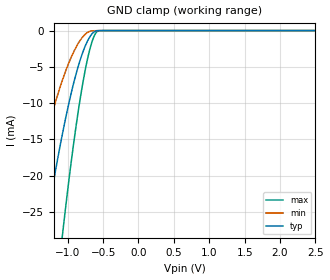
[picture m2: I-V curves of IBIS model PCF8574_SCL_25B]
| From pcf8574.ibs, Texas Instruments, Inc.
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[Model]   PCF8574_SCL_25B
Model_type  Input
Vinl=.75
Vinh=1.75
| variable   typ   min   max
C_comp   1.04pF   0.96pF   1.20pF
[Temperature Range]   40   100   -40
| Ambient temperature   25   85   -40
[Voltage range]   2.5   2.5   2.5
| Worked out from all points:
|   GND clamp passes 1 mA (typ) near -0.70 V on its own axis
[GND Clamp]
| PCF8574_SCL_25B
|   Voltage   I(typ)   I(min)   I(max)
-2.5V     -117.1mA   -74.13mA   -195.1mA
-1.63V    -48.43mA   -28.12mA   -85.63mA
-1.6V     -46.32mA   -26.75mA   -82.18mA
-1.315V   -27.58mA   -14.86mA   -51.15mA
-1.07V    -14.04mA   -6.717mA   -27.86mA
-960mV    -9.033mA   -3.902mA   -18.86mA
-870mV    -5.578mA   -2.087mA   -12.39mA
-790mV    -3.09mA    -907.2uA   -7.454mA
-710mV    -1.254mA   -201.3uA   -3.496mA
-630mV    -200.9uA   -23.45uA   -857.1uA
-560mV    -7.89uA    -10.66uA   -15.75uA
2.5V      263.9pA    417.2pA    69.6pA
